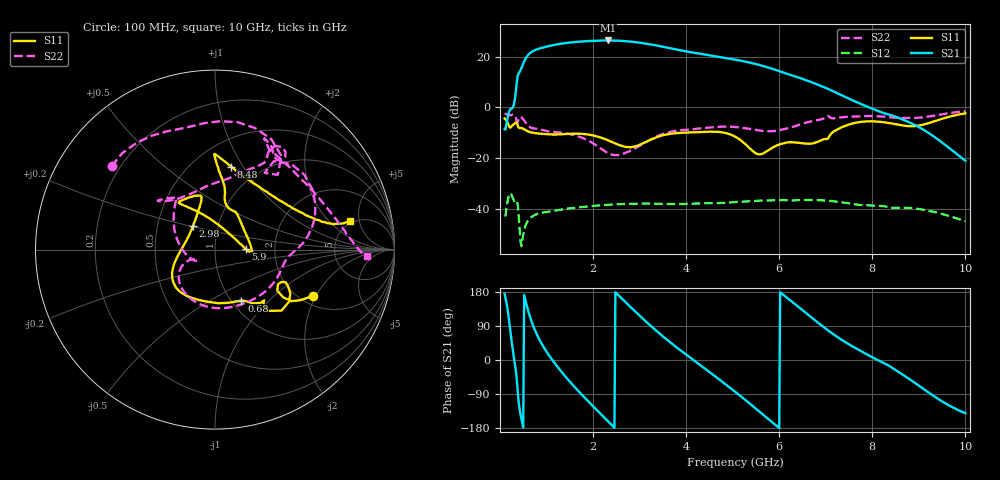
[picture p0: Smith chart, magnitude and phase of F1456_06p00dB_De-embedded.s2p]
! Integrated Device Technology
! Corporate Headquarters
! 6024 Silver Creek Valley Road
! San Jose, CA 95138  USA
! Phone:  1-408-284-8200
! Toll Free:  1-800-223-1366
! Webpage:  http://www.idt.com/
! Timing and RF Division
! 515 Groton Road, Suite 102
! Westford, MA 01886-6024
! Device:  F1456
! Description: 6-bit 0.5 dB Transmit Variable Gain Amplifier
! Frequency:  2100.0 -  2950.00 MHz
! Package:  6x6 mm Thin QFN Plastic Package: 28 pin
! State:  12
! Atten State:  6.0 dB
! Voltage:  +5.00 Volts
! Current:  217.070 mA
! Data:  The device was measured on a the F1455 evaluation board which has
!  individual transmission lines to the RF pins.  Data was collected
!  using a calibrated network analyzer.  The evaluation board was
!  de-embedded using a TRL calibration technique.
!  The reference plane is the edge of the package pin.
!  Pin  1 = CSb
!  Pin  2 = DATA
!  Pin  3 = CLK
!  Pin  4 = RSET
!  Pin  5 = GND
!  Pin  6 = RFIN  = Port 1
!  Pin  7 = GND
!  Pin  8 = NC
!  Pin  9 = NC
!  Pin 10 = NC
!  Pin 11 = NC
!  Pin 12 = NC
!  Pin 13 = NC
!  Pin 14 = /STBY
!  Pin 15 = GND
!  Pin 16 = RFOUT  = Port 2
!  Pin 17 = GND
!  Pin 18 = NC
!  Pin 19 = NC
!  Pin 20 = NC
!  Pin 21 = GND
!  Pin 22 = NC
!  Pin 23 = GND
!  Pin 24 = NC
!  Pin 25 = NC
!  Pin 26 = NC
!  Pin 27 = GND
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# GHz S dB R 50
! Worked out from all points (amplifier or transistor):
!   496 points, 100 MHz to 10 GHz, reference 50 ohm
!   highest |S21| = 26.4 dB at 2.32 GHz (marker M1)
!   |S21| within 3 dB of that: 880.1 MHz to 3.638 GHz (2.758 GHz wide, 122 % of centre)
!   unconditionally stable (mu >= 1): start of sweep to end of sweep
!   at 1.74 GHz: K = 2.13, MAG = 26.6 dB, |S12| = -39.2 dB
!   at 5.06 GHz: K = 3.37, MAG = 19.9 dB, |S12| = -37.3 dB
!   at 10 GHz: K = 114.56, MAG = -11.7 dB, |S12| = -44.8 dB
!   S11 on the Smith chart (normalised r, x): 100 MHz: 2.34, -1.90; 680 MHz: 1.11, -0.70; 2.98 GHz: 0.76, +0.21; 5.9 GHz: 1.41, +0.01; 8.48 GHz: 0.75, +0.89; 10 GHz: 4.68, +3.62
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0.1  -4.37 -25.2  -8.55 174.9  -42.47 44.4  -2.61 141.1
0.34  -5.95 -35.1  5.92 -27.1  -37.08 -143.5  -3.89 54.6
0.42  -8.10 -45.9  13.88 -128.0  -47.32 132.2  -3.89 48.2
0.56  -9.04 -56.6  19.55 151.2  -46.06 -172.2  -6.19 4.1
0.68  -9.88 -62.7  21.89 101.3  -43.13 150.1  -8.07 -9.9
0.92  -10.42 -81.2  23.58 37.8  -41.41 97.8  -8.96 -46.3
1.16  -10.65 -101.4  24.60 -5.8  -40.74 67.6  -9.64 -81.4
1.48  -10.39 -122.2  25.53 -54.2  -39.78 39.4  -10.44 -120.1
1.76  -10.40 -136.9  25.98 -91.8  -39.19 19.6  -11.92 -142.9
2.02  -11.10 -149.0  26.26 -124.6  -38.76 3.4  -14.36 -155.3
2.32  -12.96 -165.2  26.38 -161.6  -38.34 -14.1  -17.99 -154.9
2.62  -15.21 171.0  26.21 162.0  -38.07 -30.7  -18.42 -148.0
2.98  -14.88 132.4  25.56 119.4  -37.89 -49.9  -15.34 -174.8
3.4  -11.56 108.0  24.26 72.8  -37.94 -71.0  -11.20 146.3
4.1  -9.84 113.0  21.75 5.2  -37.94 -99.9  -8.69 128.3
4.6  -9.54 127.0  20.23 -40.9  -37.76 -120.8  -7.74 137.2
5.06  -11.58 120.1  18.80 -84.4  -37.31 -139.9  -7.71 139.1
5.9  -15.39 1.6  14.94 -169.4  -36.57 175.8  -9.28 105.5
6.7  -14.23 31.0  9.90 111.4  -36.46 127.9  -5.44 62.0
8.36  -6.13 83.7  -2.81 -15.4  -39.34 49.7  -3.86 62.6
8.48  -6.54 79.0  -3.52 -24.8  -39.52 47.1  -3.97 60.2
10  -2.31 12.0  -20.97 -140.4  -44.76 -32.4  -1.46 -2.5
